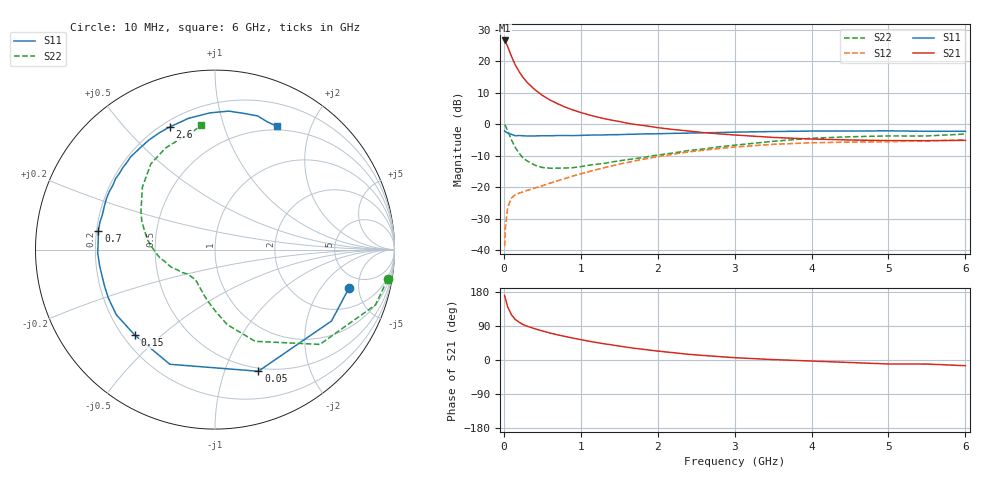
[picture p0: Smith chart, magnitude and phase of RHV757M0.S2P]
! SIEMENS Small Signal Semiconductors
! BFR106
! Si NPN RF Bipolar Junction Transistor in SOT23
! VCE = 0.75 V  IC = 7 mA
! Common Emitter S-Parameters:  August  1996
# GHz  S  MA  R  50
!  f  S11  S21  S12  S22
! GHz  MAG  ANG  MAG  ANG  MAG  ANG  MAG  ANG
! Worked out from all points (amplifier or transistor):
!   36 points, 10 MHz to 6 GHz, reference 50 ohm
!   highest |S21| = 26.5 dB at 10 MHz (marker M1)
!   |S21| within 3 dB of that: start of sweep to 66.84 MHz
!   unconditionally stable (mu >= 1): 514.6 MHz to end of sweep
!   at 250 MHz: K = 0.62, MSG = 18.1 dB, |S12| = -21.5 dB
!   at 1.4 GHz: K = 1.16, MAG = 4.8 dB, |S12| = -13.3 dB
!   at 6 GHz: K = 1.03, MAG = -1.1 dB, |S12| = -5.0 dB
!   S11 on the Smith chart (normalised r, x): 10 MHz: 3.61, -3.89; 50 MHz: 0.47, -1.31; 150 MHz: 0.25, -0.41; 700 MHz: 0.21, +0.08; 2.6 GHz: 0.23, +0.67; 6 GHz: 0.45, +1.52
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0.01  0.7766 -16.0  21.2 170.2  0.0116 83.5  0.9759 -9.7
0.02  0.7613 -31.5  20.44 162.1  0.0229 74.7  0.9458 -19.0
0.05  0.7195 -70.4  16.93 140.1  0.048 57.2  0.7878 -42.1
0.1  0.6866 -111.5  11.83 119.1  0.0677 41.9  0.5576 -66.4
0.15  0.653 -133.3  8.612 106.7  0.0757 36.3  0.4237 -80.7
0.2  0.6589 -146.6  6.761 99.4  0.0805 35.1  0.3429 -89.6
0.25  0.6526 -155.7  5.482 93.6  0.0845 34.8  0.2907 -97.7
0.3  0.6481 -161.9  4.623 89.5  0.0886 35.9  0.2625 -103.2
0.4  0.649 -171.9  3.542 82.6  0.0966 38.6  0.224 -112.9
0.5  0.6538 -178.3  2.859 76.7  0.1053 41.7  0.2052 -120.0
0.6  0.6525 175.7  2.411 71.2  0.1158 44.2  0.1998 -124.8
0.7  0.6585 170.8  2.101 66.3  0.1262 46.4  0.2002 -129.7
0.9  0.657 162.5  1.673 57.7  0.1504 49.2  0.2037 -138.2
1.1  0.6686 154.6  1.408 49.8  0.1757 50.5  0.2222 -144.9
1.3  0.6727 147.7  1.224 42.9  0.203 50.7  0.2381 -151.8
1.6  0.6876 138.3  1.036 33.8  0.2456 49.3  0.2723 -161.5
2.2  0.7131 121.0  0.821 19.3  0.3336 42.6  0.3481 178.6
2.6  0.7288 110.2  0.732 11.9  0.3868 36.3  0.4042 165.5
3.5  0.7623 92.1  0.615 1.1  0.4779 21.3  0.5336 139.3
4.5  0.7757 77.9  0.56 -6.6  0.5186 5.9  0.6294 116.0
5.5  0.7687 67.5  0.546 -10.7  0.5433 -3.2  0.6489 104.6
6  0.769 63.5  0.553 -15.1  0.5592 -9.7  0.696 96.4
